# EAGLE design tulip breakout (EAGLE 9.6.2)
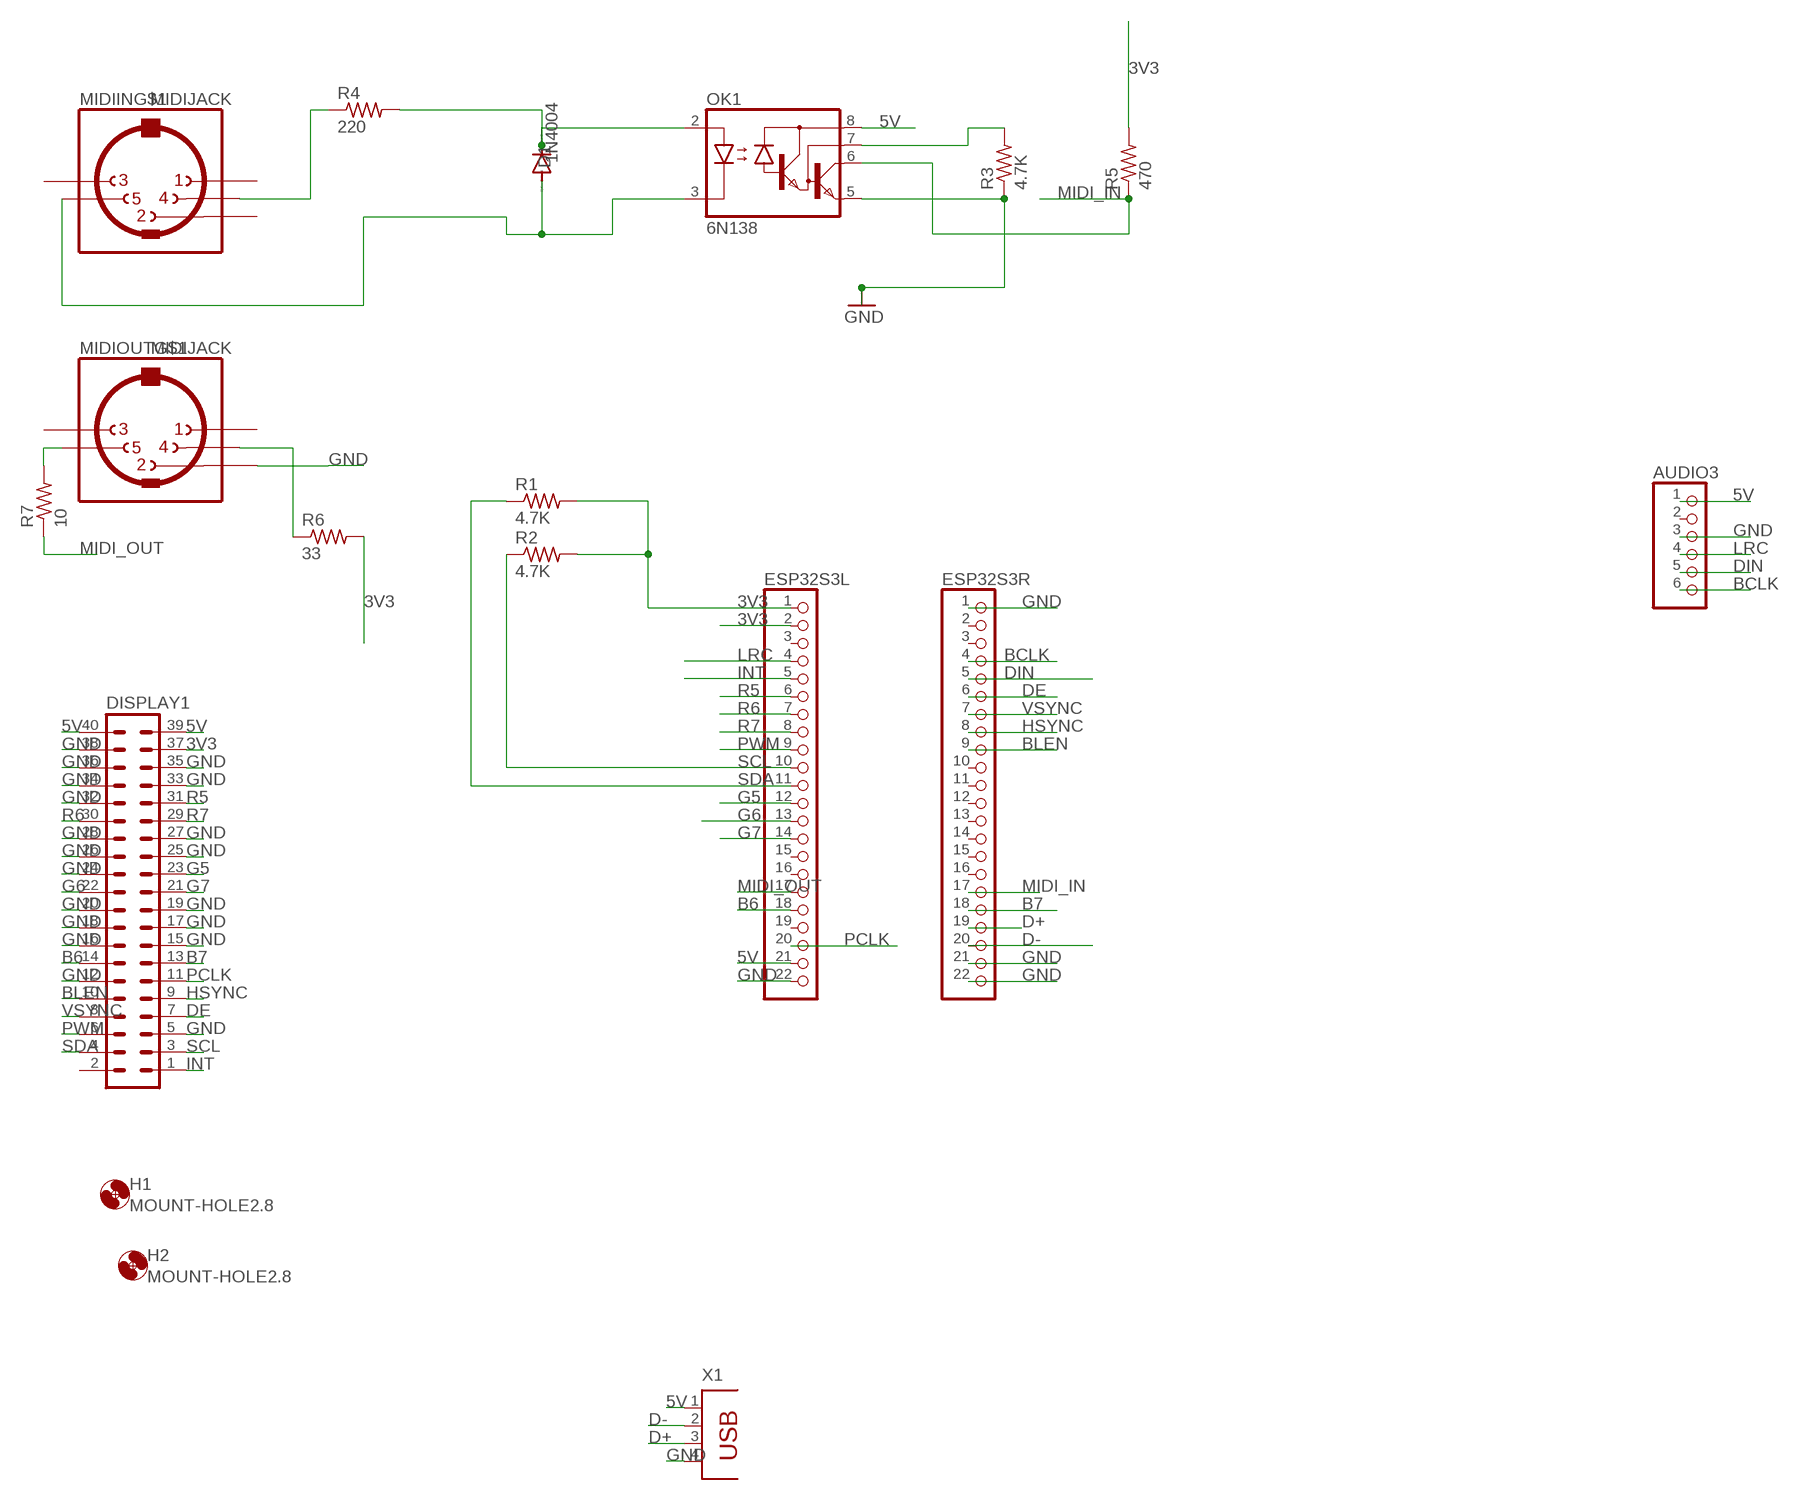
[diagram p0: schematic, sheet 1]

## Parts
AUDIO3  PINHD-1X6  [1X06]
D1  1N4004  [DO41-10]
DISPLAY1  MA20-2  [MA20-2]
ESP32S3L  PINHD-1X22  [1X22]
ESP32S3R  PINHD-1X22  [1X22]
H1  MOUNT-HOLE2.8  [2,8]
H2  MOUNT-HOLE2.8  [2,8]
MIDIIN  MIDIJACK  [CP-2350]
MIDIOUT  MIDIJACK  [CP-2350]
OK1  6N138  [DIL08]
R1  4.7K  R-US_0207/12  [0207/12]
R2  4.7K  R-US_0207/12  [0207/12]
R3  4.7K  R-US_0207/12  [0207/12]
R4  220  R-US_0207/12  [0207/12]
R5  470  R-US_0207/12  [0207/12]
R6  33  R-US_0207/12  [0207/12]
R7  10  R-US_0207/12  [0207/12]
X1  PN87520  [PN87520]

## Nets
3V3: DISPLAY1.37 ESP32S3L.1 ESP32S3L.2 R1.2 R2.2 R5.2 R6.2
5V: AUDIO3.1 DISPLAY1.39 DISPLAY1.40 ESP32S3L.21 OK1.8(VCC) X1.1
B6: DISPLAY1.14 ESP32S3L.18
B7: DISPLAY1.13 ESP32S3R.18
BCLK: AUDIO3.6 ESP32S3R.4
BLEN: DISPLAY1.10 ESP32S3R.9
D+: ESP32S3R.19 X1.3
D-: ESP32S3R.20 X1.2
DE: DISPLAY1.7 ESP32S3R.6
DIN: AUDIO3.5 ESP32S3R.5
G5: DISPLAY1.23 ESP32S3L.12
G6: DISPLAY1.22 ESP32S3L.13
G7: DISPLAY1.21 ESP32S3L.14
GND: AUDIO3.3 DISPLAY1.5 DISPLAY1.12 DISPLAY1.15 DISPLAY1.16 DISPLAY1.17 DISPLAY1.18 DISPLAY1.19 DISPLAY1.20 DISPLAY1.24 DISPLAY1.25 DISPLAY1.26 DISPLAY1.27 DISPLAY1.28 DISPLAY1.32 DISPLAY1.33 DISPLAY1.34 DISPLAY1.35 DISPLAY1.36 DISPLAY1.38 ESP32S3L.22 ESP32S3R.1 ESP32S3R.21 ESP32S3R.22 MIDIOUT.2 OK1.5(GND) R3.1 X1.4
HSYNC: DISPLAY1.9 ESP32S3R.8
INT: DISPLAY1.1 ESP32S3L.5
LRC: AUDIO3.4 ESP32S3L.4
MIDI_IN: ESP32S3R.17 OK1.6(VO) R5.1
MIDI_OUT: ESP32S3L.17 R7.1
N$29: MIDIIN.4 R4.1
N$30: D1.C OK1.2(A) R4.2
N$31: D1.A MIDIIN.5 OK1.3(C)
N$32: OK1.7(VB) R3.2
N$34: MIDIOUT.5 R7.2
N$35: MIDIOUT.4 R6.1
PCLK: DISPLAY1.11 ESP32S3L.20
PWM: DISPLAY1.6 ESP32S3L.9
R5: DISPLAY1.31 ESP32S3L.6
R6: DISPLAY1.30 ESP32S3L.7
R7: DISPLAY1.29 ESP32S3L.8
SCL: DISPLAY1.3 ESP32S3L.10 R2.1
SDA: DISPLAY1.4 ESP32S3L.11 R1.1
VSYNC: DISPLAY1.8 ESP32S3R.7
Unconnected: AUDIO3.2 DISPLAY1.2 ESP32S3L.3 ESP32S3L.15 ESP32S3L.16 ESP32S3L.19 ESP32S3R.2 ESP32S3R.3 ESP32S3R.10 ESP32S3R.11 ESP32S3R.12 ESP32S3R.13 ESP32S3R.14 ESP32S3R.15 ESP32S3R.16 MIDIIN.1 MIDIIN.2 MIDIIN.3 MIDIIN.PE1(MT) MIDIIN.PE2(MT) MIDIIN.PE(MT) MIDIIN.PE@(MT) MIDIOUT.1 MIDIOUT.3 MIDIOUT.PE1(MT) MIDIOUT.PE2(MT) MIDIOUT.PE(MT) MIDIOUT.PE@(MT)

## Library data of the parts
AUDIO3 = pinhead:PINHD-1X6: PIN HEADER
D1 = diode:1N4004: DIODE
DISPLAY1 = con-lstb:MA20-2: PIN HEADER; OC_FARNELL: unknown; OC_NEWARK: unknown
ESP32S3L ESP32S3R = pinhead:PINHD-1X22: PIN HEADER
H1 H2 = holes:MOUNT-HOLE: MOUNTING HOLE with drill center marker
MIDIIN MIDIOUT = adafruit:MIDIJACK: DIN 5 jack also known as MIDI jack A modification of conn-hirshman:MAB5SH with two options for the grounding 'teeth'
OK1 = optocoupler:6N138: MOTOROLA OPTO COUPLER; MF: VISHAY/TELEFUNKEN; MPN: 6N138; OC_FARNELL: 9860150; OC_NEWARK: 35K5294
R1-R7 = rcl:R-US_: RESISTOR, American symbol; SPICEPREFIX: R
X1 = con-berg:PN87520: BERG USB connector; OC_FARNELL: unknown; OC_NEWARK: unknown

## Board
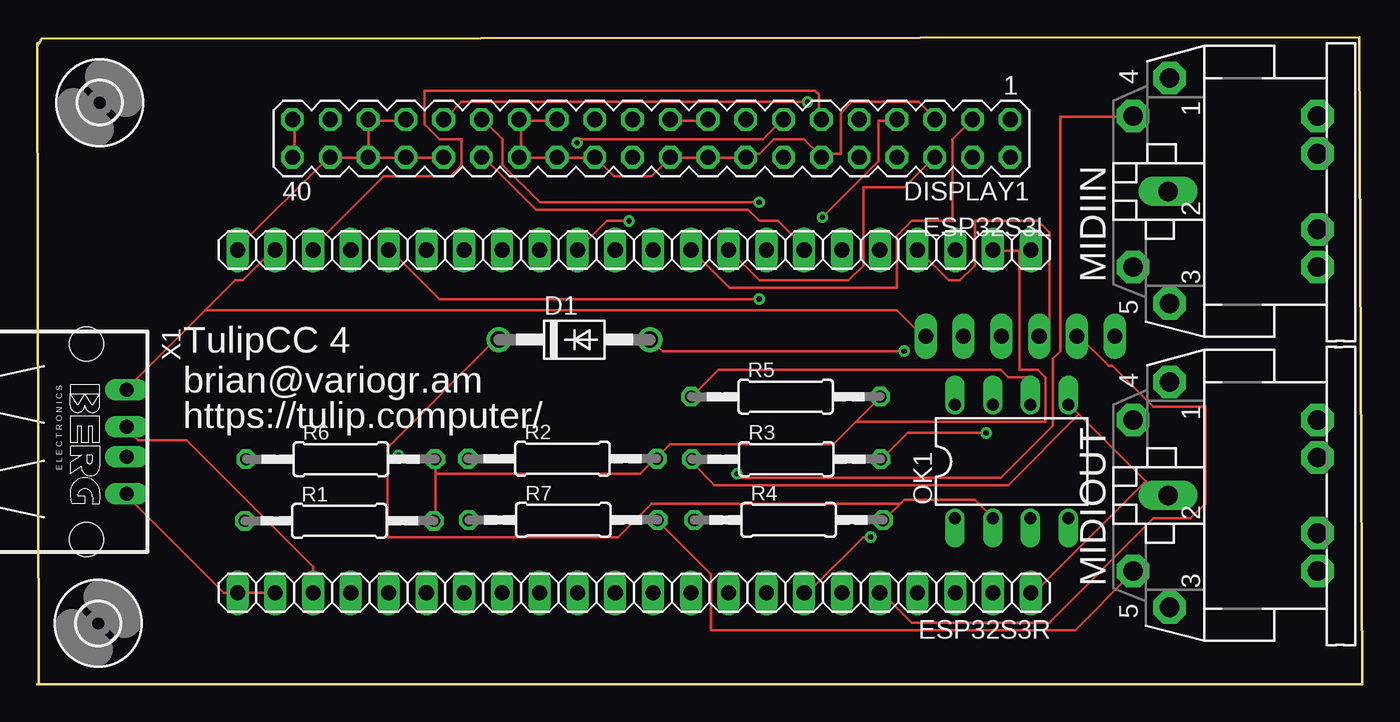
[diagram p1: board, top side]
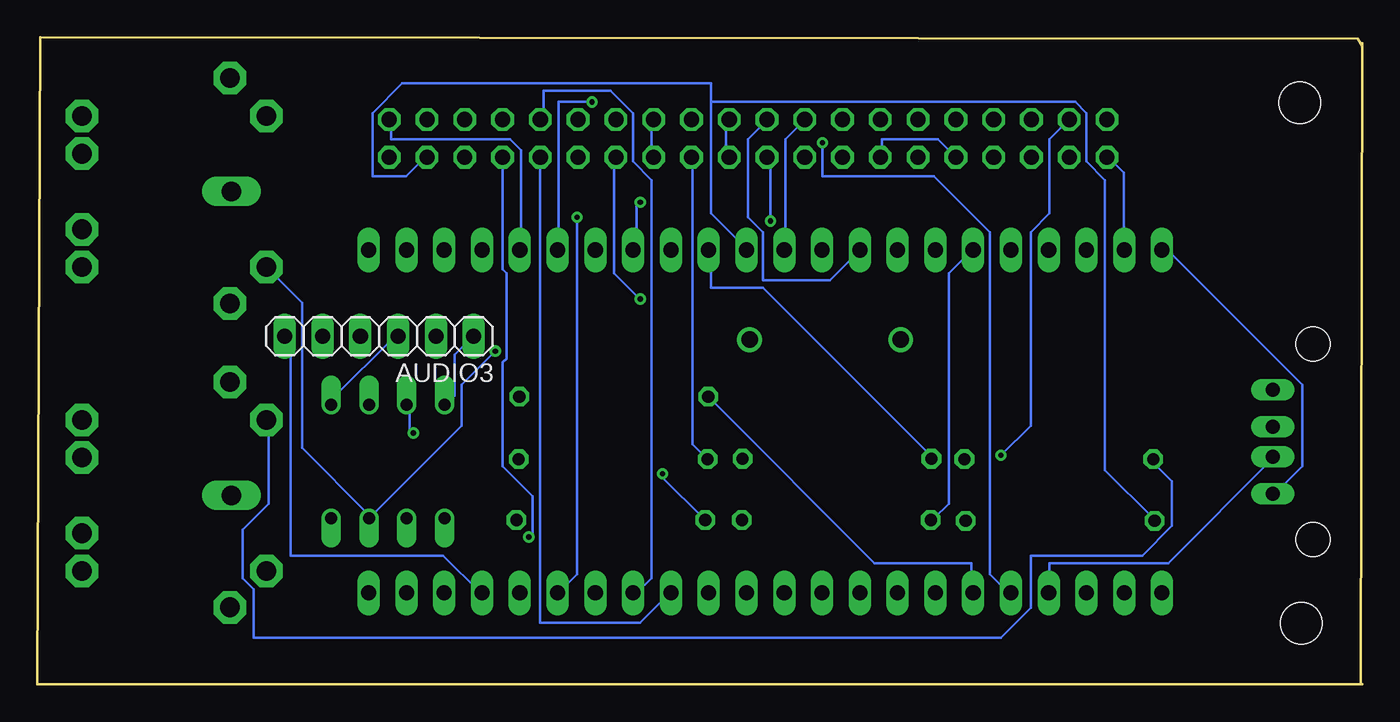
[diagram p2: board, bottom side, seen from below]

Size 89.1 x 43.5 mm. Coordinates in mm from the lower left corner, seen from the top.
Outline: 0,43.1 0,42.9
Outline: 0,42.9 0.1,0
Outline: 0,42.9 0.3,43.4 88.9,43.5 89.1,0 0,0
Copper layers (1*16): Top 0.035mm / dielectric 0.15mm / Bottom 0.035mm
Design rules "default *": minimum track width 6mil, minimum drill 0.35mm, track to track 10mil, track to pad 10mil, pad to pad 10mil, via to via 10mil, smd to smd 10mil, copper to edge 40mil, drill to drill 6mil, minimum pad ring 10mil, minimum via ring 8mil, stop-mask expansion 4mil, vias tented up to drill 0mil, thermal gap 10mil

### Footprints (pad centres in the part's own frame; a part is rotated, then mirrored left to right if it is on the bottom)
1X06 = drill 1.016 long: 1 -6.35,0; 2 -3.81,0; 3 -1.27,0; 4 1.27,0; 5 3.81,0; 6 6.35,0
DO41-10 = drill 1.118: A 5.08,0; C -5.08,0
MA20-2 = drill 1.016 octagon: 1 -24.13,-1.27; 2 -24.13,1.27; 3 -21.59,-1.27; 4 -21.59,1.27; 5 -19.05,-1.27; 6 -19.05,1.27; 7 -16.51,-1.27; 8 -16.51,1.27; 9 -13.97,-1.27; 10 -13.97,1.27; 11 -11.43,-1.27; 12 -11.43,1.27; 13 -8.89,-1.27; 14 -8.89,1.27; 15 -6.35,-1.27; 16 -6.35,1.27; 17 -3.81,-1.27; 18 -3.81,1.27; 19 -1.27,-1.27; 20 -1.27,1.27; 21 1.27,-1.27; 22 1.27,1.27; 23 3.81,-1.27; 24 3.81,1.27; 25 6.35,-1.27; 26 6.35,1.27; 27 8.89,-1.27; 28 8.89,1.27; 29 11.43,-1.27; 30 11.43,1.27; 31 13.97,-1.27; 32 13.97,1.27; 33 16.51,-1.27; 34 16.51,1.27; 35 19.05,-1.27; 36 19.05,1.27; 37 21.59,-1.27; 38 21.59,1.27; 39 24.13,-1.27; 40 24.13,1.27
1X22 = drill 1.016 long: 1 -26.67,0; 2 -24.13,0; 3 -21.59,0; 4 -19.05,0; 5 -16.51,0; 6 -13.97,0; 7 -11.43,0; 8 -8.89,0; 9 -6.35,0; 10 -3.81,0; 11 -1.27,0; 12 1.27,0; 13 3.81,0; 14 6.35,0; 15 8.89,0; 16 11.43,0; 17 13.97,0; 18 16.51,0; 19 19.05,0; 20 21.59,0; 21 24.13,0; 22 26.67,0
2,8 = hole 2.8: 0,0
CP-2350 = drill 1.321 pad 2.184 octagon: 1 7.62,12.58; 3 -7.52,12.58; 4 5.08,15.02; 5 -5.08,15.02; PE -2.54,2.62; PE1 -5.08,2.62; PE2 5.08,2.62; PE@ 2.54,2.62 | drill 1.321 long: 2 0,12.68
DIL08 = drill 0.813 offset: 1 -3.81,-3.81; 2 -1.27,-3.81; 3 1.27,-3.81; 4 3.81,-3.81; 5 3.81,3.81; 6 1.27,3.81; 7 -1.27,3.81; 8 -3.81,3.81
0207/12 = drill 0.813 octagon: 1 -6.35,0; 2 6.35,0
PN87520 = drill 0.95 long: 1 -3.5,2.71; 2 -1,2.71; 3 1,2.71; 4 3.5,2.71 | hole 2.3: -6.57,0; 6.57,0

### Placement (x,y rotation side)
AUDIO3  66.1,23.4 180 bottom
D1  36.12,23.17 0 top
DISPLAY1  41.3,36.7 180 top
ESP32S3L  40.14,29.2 180 top
ESP32S3R  40.14,6.15 180 top
H1  4.1,4.1 0 top
H2  4.2,39.1 0 top
MIDIIN  88.71,33.13 90 top
MIDIOUT  88.71,12.7 90 top
OK1  65.52,14.98 0 top
R1  20.32,10.99 0 top
R2  35.32,15.17 0 top
R3  50.37,15.14 0 top
R4  50.53,11.05 0 top
R5  50.33,19.34 0 top
R6  20.41,15.14 0 top
R7  35.37,11.05 0 top
X1  3.31,16.31 270 top

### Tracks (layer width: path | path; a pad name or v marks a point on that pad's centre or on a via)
3V3  (via drill 0.35)
  Top 0.152: 66.05,29.15 66.8,29.15 ESP32S3L.1 66.05,29.15 | 66.05,29.15 64.3,29.15 ESP32S3L.2 | 26.8,14.15 26.8,14.9 R6.2 26.55,15.15 24.55,15.15 v24.3,15.4 | 26.8,14.15 26.8,11.15 R1.2 | 26.8,14.15 40.55,14.15 41.55,15.15 R2.2 41.8,15.4 42.55,16.15 53.55,16.15 55.05,17.65 | 55.05,17.65 56.55,19.15 R5.2 | 66.05,29.15 66.05,21.15 67.3,21.15 67.8,20.65 67.8,17.65 55.05,17.65
  Bottom 0.152: v24.3,15.4 22.3,17.4 22.3,30.4 21.05,31.65 21.05,36.65 19.8,37.9 DISPLAY1.37
5V
  Top 0.152: DISPLAY1.40 17.3,35.65 17.3,37.9 DISPLAY1.39 | 11.3,25.15 13.3,27.15 13.8,27.15 15.8,29.15 ESP32S3L.21 | 11.3,25.15 6.05,19.9 X1.1 | 11.3,25.15 57.8,25.15 59.55,23.4 AUDIO3.1
  Bottom 0.152: OK1.8 61.55,18.9 61.05,19.4 61.05,22.15 59.8,23.4 AUDIO3.1 | DISPLAY1.40 17.05,35.4 16.05,34.4 16.05,29.4 ESP32S3L.21
B6  (via drill 0.35)
  Top 0.152: v48.55,25.9 27.05,25.9 23.8,29.15 ESP32S3L.18
  Bottom 0.152: v48.55,25.9 50.3,27.65 50.3,35.4 DISPLAY1.14
B7  (via drill 0.35)
  Top 0.152: v36.3,36.4 36.55,36.65 48.8,36.65 50.05,37.9 DISPLAY1.13
  Bottom 0.152: v36.3,36.4 36.3,34.15 28.8,34.15 25.05,30.4 25.05,7.4 23.8,6.15 ESP32S3R.18
BCLK
  Bottom 0.152: ESP32S3R.4 59.3,6.15 61.8,8.65 72.05,8.65 72.05,23.15 72.3,23.4 AUDIO3.6
BLEN
  Bottom 0.152: ESP32S3R.9 46.55,6.15 48.55,4.15 55.3,4.15 55.3,35.4 DISPLAY1.10
D+
  Bottom 0.152: X1.3 6.05,15.15 13.05,8.15 21.05,8.15 21.05,6.15 ESP32S3R.19
D-
  Top 0.152: ESP32S3R.20 18.55,7.9 10.05,16.4 6.8,16.4 6.05,17.15 X1.2
DE  (via drill 0.35)
  Top 0.152: v52.8,31.4 56.55,35.15 56.55,37.9 57.8,37.9 DISPLAY1.7
  Bottom 0.152: v52.8,31.4 52.8,7.4 54.05,6.15 ESP32S3R.6
DIN
  Top 0.152: ESP32S3R.5 56.8,6.15 58.8,4.15 68.05,4.15 75.05,11.15 77.55,11.15 78.55,12.15 78.55,18.65 75.05,18.65 72.3,21.4 72.05,21.4 70.05,23.4 AUDIO3.5
G5
  Bottom 0.152: ESP32S3L.12 38.8,29.4 38.8,36.65 37.55,37.9 DISPLAY1.23
G6  (via drill 0.35)
  Top 0.152: v39.8,31.15 38.3,31.15 36.55,29.4 ESP32S3L.13
  Bottom 0.152: v39.8,31.15 39.8,35.4 DISPLAY1.22
G7
  Bottom 0.152: ESP32S3L.14 33.8,29.15 35.8,27.15 40.3,27.15 40.3,30.4 41.3,31.4 41.3,36.65 40.05,37.9 DISPLAY1.21
GND
  Top 0.152: X1.4 6.05,12.65 12.55,6.15 ESP32S3R.22 ESP32S3R.21 | 22.3,37.9 24.55,37.9 DISPLAY1.33 | DISPLAY1.36 22.3,35.4 24.55,35.4 DISPLAY1.34 24.8,35.4 27.3,35.4 DISPLAY1.32 | 22.3,37.9 22.3,35.65 DISPLAY1.36 | 22.3,37.9 DISPLAY1.35 | ESP32S3L.22 13.55,29.4 19.55,35.4 DISPLAY1.38 19.8,35.4 22.05,35.4 DISPLAY1.36 | 74.55,13.65 75.3,12.9 75.8,12.9 MIDIOUT.2 | 74.55,13.65 70.05,18.15 | 70.05,18.15 69.55,18.65 OK1.5 | 74.55,13.65 67.05,6.15 ESP32S3R.1 | 32.55,37.9 34.8,37.9 DISPLAY1.25 | 32.55,37.9 32.55,35.65 DISPLAY1.28 32.55,35.4 34.8,35.4 DISPLAY1.26 35.05,35.4 37.3,35.4 DISPLAY1.24 37.55,35.4 38.8,34.15 41.3,34.15 42.55,35.4 DISPLAY1.20 42.8,35.4 45.05,35.4 DISPLAY1.18 45.3,35.4 47.55,35.4 DISPLAY1.16 47.8,35.65 48.55,35.65 49.55,36.65 51.55,36.65 52.55,35.65 DISPLAY1.12 52.8,35.65 54.05,35.65 54.05,38.4 54.8,39.15 59.3,39.15 60.3,38.15 DISPLAY1.5 | 32.55,37.9 DISPLAY1.27 | DISPLAY1.19 42.8,37.9 45.05,37.9 DISPLAY1.17 | 70.05,18.15 65.3,13.4 45.55,13.4 44.05,14.9 R3.1
  Bottom 0.152: X1.4 5.8,12.9 4.05,14.65 4.05,20.15 13.3,29.4 ESP32S3L.22 | AUDIO3.3 65.05,23.4 69.3,19.15 69.3,18.9 OK1.5 | R3.1 44.05,15.15 45.05,16.15 45.05,35.4 DISPLAY1.18 | DISPLAY1.15 47.8,37.9 47.8,35.65 DISPLAY1.16 | DISPLAY1.19 42.8,37.9 42.8,35.65 DISPLAY1.20 | DISPLAY1.32 28.55,36.65 32.3,36.65 32.3,35.65 DISPLAY1.28
HSYNC
  Bottom 0.152: ESP32S3R.8 48.8,6.15 47.8,7.15 47.8,33.9 49.05,35.15 49.05,38.4 50.55,39.9 55.05,39.9 55.05,38.15 DISPLAY1.9
INT
  Bottom 0.152: ESP32S3L.5 56.55,29.4 56.55,35.9 57.3,36.65 65.3,36.65 65.3,37.9 DISPLAY1.1
LRC
  Top 0.152: AUDIO3.4 68.05,23.4 68.05,30.4 67.3,31.15 63.05,31.15 63.05,28.15 62.05,27.15 61.3,27.15 59.3,29.15 ESP32S3L.4
MIDI_IN
  Top 0.152: OK1.6 66.55,18.9 66.55,20.65 65.3,20.65 64.8,21.15 45.8,21.15 44.05,19.4 R5.1
  Bottom 0.152: R5.1 43.8,19.15 32.8,8.15 26.3,8.15 26.3,6.15 ESP32S3R.17
MIDI_OUT
  Bottom 0.152: R7.1 28.8,11.15 27.8,12.15 27.8,27.65 26.3,29.15 ESP32S3L.17
N$29  (via drill 0.35)
  Top 0.152: v47.05,14.15 47.3,13.9 64.8,13.9 68.3,17.4 68.3,21.9 68.8,22.4 68.8,38.15 73.55,38.15 MIDIIN.4
  Bottom 0.152: v47.05,14.15 47.05,13.9 44.3,11.15 R4.1
N$30
  Top 0.152: 58.05,12.15 58.3,12.4 63.05,12.4 64.05,11.4 OK1.2 | 58.05,12.15 57.05,11.15 R4.2 | 58.05,12.15 41.3,12.15 39.05,9.9 23.55,9.9 23.55,15.9 30.8,23.15 D1.C
N$31  (via drill 0.35)
  Top 0.152: v58.3,22.4 42.05,22.4 41.3,23.15 D1.A
  Bottom 0.152: MIDIIN.5 73.55,27.9 71.3,25.65 71.3,15.9 66.8,11.4 OK1.3 66.55,11.4 60.55,17.4 60.55,20.15 v58.3,22.4
N$32  (via drill 0.35)
  Top 0.152: v63.8,16.9 58.55,16.9 56.8,15.15 R3.2
  Bottom 0.152: v63.8,16.9 64.05,17.15 64.05,18.65 OK1.7
N$34
  Top 0.152: R7.2 41.8,10.9 45.3,7.4 45.3,3.65 69.8,3.65 73.55,7.4 MIDIOUT.5
N$35
  Bottom 0.152: R6.1 14.05,14.9 12.8,13.65 12.8,10.65 14.8,8.65 22.3,8.65 22.3,5.15 24.3,3.15 74.55,3.15 74.55,6.4 75.3,7.15 75.3,10.4 73.55,12.15 73.55,17.65 MIDIOUT.4
PCLK
  Top 0.152: ESP32S3L.20 18.55,29.4 23.3,34.15 27.8,34.15 28.55,34.9 28.55,36.65 27.05,36.65 26.05,37.65 26.05,39.9 52.3,39.9 52.55,39.65 52.55,38.15 DISPLAY1.11
PWM
  Top 0.152: ESP32S3L.9 46.55,29.15 48.55,27.15 54.55,27.15 55.55,28.15 55.55,33.4 58.3,33.4 60.3,35.4 DISPLAY1.6
R5  (via drill 0.35)
  Top 0.152: v51.8,39.15 28.55,39.15 27.55,38.15 DISPLAY1.31
  Bottom 0.152: v51.8,39.15 54.05,39.15 54.05,29.4 ESP32S3L.6
R6
  Top 0.152: DISPLAY1.30 30.05,35.4 33.55,31.9 47.8,31.9 48.55,31.15 49.8,31.15 51.55,29.4 ESP32S3L.7
R7  (via drill 0.35)
  Top 0.152: v48.55,32.4 33.8,32.4 31.3,34.9 31.3,36.65 30.05,37.9 DISPLAY1.29
  Bottom 0.152: v48.55,32.4 48.8,32.15 48.8,29.4 ESP32S3L.8
SCL
  Top 0.152: DISPLAY1.3 62.8,37.9 61.55,36.65 61.55,31.15 58.8,31.15 57.8,30.15 57.8,26.65 46.55,26.65 44.05,29.15 ESP32S3L.10
  Bottom 0.152: R2.1 29.05,15.4 40.3,26.65 43.8,26.65 43.8,29.15 ESP32S3L.10
SDA
  Bottom 0.152: 43.8,39.15 19.3,39.15 18.55,38.4 18.55,35.15 17.3,33.9 17.3,14.4 14.05,11.15 R1.1 | 43.8,39.15 43.8,31.65 41.55,29.4 ESP32S3L.11 | 43.8,39.15 43.8,40.4 64.55,40.4 66.55,38.4 66.55,34.15 64.3,34.15 63.05,35.4 DISPLAY1.4
VSYNC  (via drill 0.35)
  Top 0.152: v56.05,9.9 55.55,9.9 51.8,6.15 ESP32S3R.7
  Bottom 0.152: v56.05,9.9 55.8,10.15 55.8,12.65 57.8,14.65 57.8,21.65 57.55,21.9 57.55,27.65 57.8,27.9 57.8,35.4 DISPLAY1.8

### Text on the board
tPlace: TulipCC 4 / brian@variogr.am | https://tulip.computer/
